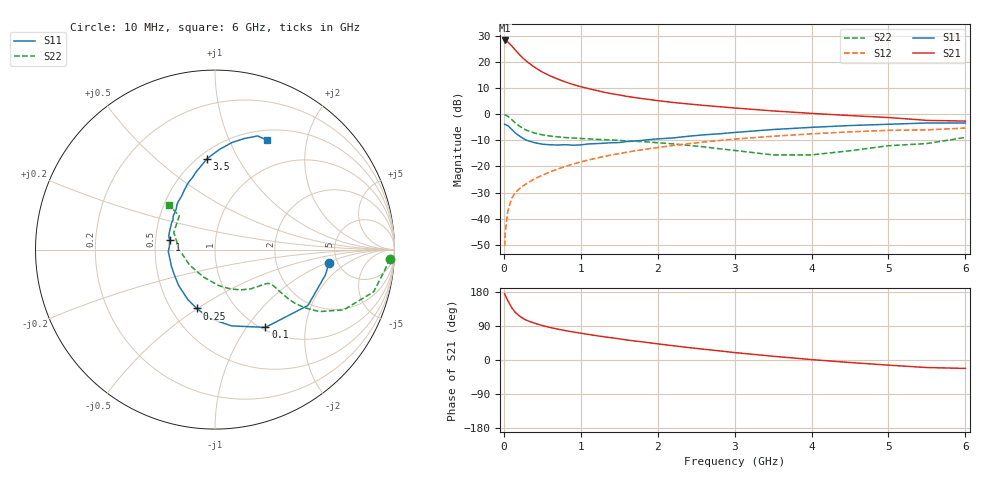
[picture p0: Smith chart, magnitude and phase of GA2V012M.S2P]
! Infineon Technologies  Discrete & RF Semiconductors
! BF775
! Si NPN RF Bipolar Junction Transistor in SOT23
! VCE = 2 V  IC = 12 mA
! Common Emitter S-Parameters:  May  1996
# GHz  S  MA  R  50
!  f  S11  S21  S12  S22
! GHz  MAG  ANG  MAG  ANG  MAG  ANG  MAG  ANG
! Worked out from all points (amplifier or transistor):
!   36 points, 10 MHz to 6 GHz, reference 50 ohm
!   highest |S21| = 28.1 dB at 10 MHz (marker M1)
!   |S21| within 3 dB of that: start of sweep to 129.2 MHz
!   unconditionally stable (mu >= 1): 473.8 MHz to 3.726 GHz
!   at 250 MHz: K = 0.76, MSG = 24.4 dB, |S12| = -27.4 dB
!   at 1.4 GHz: K = 1.13, MAG = 9.5 dB, |S12| = -15.6 dB
!   at 6 GHz: K = 0.98, MSG = 1.3 dB, |S12| = -5.3 dB
!   S11 on the Smith chart (normalised r, x): 10 MHz: 4.28, -1.05; 100 MHz: 1.04, -1.23; 250 MHz: 0.67, -0.50; 1 GHz: 0.59, +0.07; 3.5 GHz: 0.55, +0.75; 6 GHz: 0.62, +1.39
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0.01  0.6399 -6.5  25.54 175.2  0.003 86.2  0.9746 -3.0
0.02  0.6312 -12.9  25.4 170.1  0.0057 80.5  0.9571 -6.2
0.05  0.6042 -31.0  23.98 157.0  0.0137 77.4  0.9147 -14.9
0.1  0.5165 -57.0  20.27 139.0  0.0244 67.5  0.7916 -25.1
0.15  0.4352 -77.7  16.67 125.4  0.0317 63.2  0.6764 -30.7
0.2  0.385 -93.9  13.86 116.6  0.0373 62.0  0.5938 -33.0
0.25  0.3434 -107.3  11.68 109.6  0.0426 61.2  0.5329 -33.9
0.3  0.3158 -118.9  10.07 104.4  0.0474 62.4  0.4883 -33.8
0.4  0.2844 -135.5  7.848 97.1  0.0582 63.2  0.4341 -33.0
0.5  0.2659 -149.3  6.359 90.9  0.0678 64.3  0.4017 -32.2
0.6  0.2596 -159.9  5.393 85.9  0.0786 65.0  0.3817 -31.8
0.7  0.2567 -168.9  4.674 81.5  0.0893 65.2  0.368 -31.9
0.8  0.2604 -177.6  4.112 77.6  0.1003 65.0  0.3568 -32.1
1  0.2582 168.4  3.343 70.7  0.122 64.3  0.3427 -33.6
1.1  0.2693 163.4  3.071 67.5  0.1329 63.8  0.3366 -35.0
1.3  0.2779 152.8  2.628 61.4  0.155 62.3  0.325 -37.5
1.6  0.2992 140.9  2.183 52.8  0.1872 59.5  0.308 -42.7
2.2  0.3504 122.2  1.67 37.7  0.2513 52.8  0.2699 -56.0
3.5  0.5081 95.0  1.151 9.9  0.378 35.6  0.1661 -112.5
4.5  0.6051 80.8  0.938 -6.6  0.4583 22.0  0.1996 179.8
5.5  0.6764 69.4  0.759 -19.9  0.5001 7.6  0.2741 136.5
6  0.6751 64.6  0.736 -22.2  0.5415 3.6  0.359 136.1
